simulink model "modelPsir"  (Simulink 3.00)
settings: Solver=ode45  SolverMode=SingleTasking  StartTime=0.0  StopTime=0..5  MaxStep=0.0001  RelTol=1e-5  AbsTol=1e-5
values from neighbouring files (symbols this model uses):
  J = 0.0017    [Data.m]
  kr = Lm/Lr    (= 0.963591022444)    [Data.m]
  Lm = .5796    (= 0.5796)    [Data.m]
  Ls1 = Ls-Lm^2/Lr    (= 0.0430026433915)    [Data.m]
  p = 1    [Data.m]
  R1 = Rs+kr^2*Rr    (= 11.0434783366)    [Data.m]
  T1 = Ls1/R1    (= 0.00389394012293)    [Data.m]
  Tr = Lr/Rr    (= 0.162567567568)    [Data.m]
libraries: simulink_extras x1

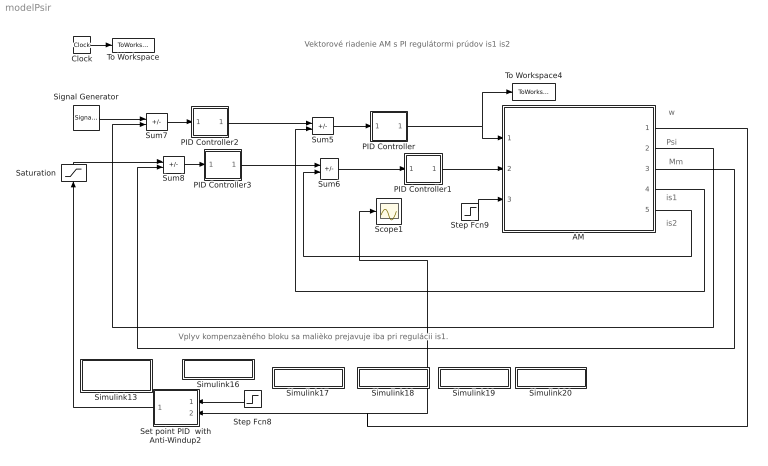
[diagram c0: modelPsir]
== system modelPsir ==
  note: w
  note: Psi
  note: Mm
  note: is1
  note: is2
  note: Vektorové riadenie AM s PI regulátormi prúdov is1 is2
  note: Vplyv kompenzaèného bloku sa malièko prejavuje iba pri regulácii is1.
  AM : Subsystem
  Clock : Clock
  PID Controller : Subsystem  mask(PID Controller){}
      mask help: Enter expressions for proportional, integral, and derivative terms. P+I/s+Ds
      mask init:
      | P=@1; I=@2; D=@3;
  PID Controller1 : Subsystem  mask(PID Controller){}
      mask help: Enter expressions for proportional, integral, and derivative terms. P+I/s+Ds
      mask init:
      | P=@1; I=@2; D=@3;
  PID Controller2 : Subsystem  mask(PID Controller){}
      mask help: Enter expressions for proportional, integral, and derivative terms. P+I/s+Ds
      mask init:
      | P=@1; I=@2; D=@3;
  PID Controller3 : Subsystem  mask(PID Controller){}
      mask help: Enter expressions for proportional, integral, and derivative terms. P+I/s+Ds
      mask init:
      | P=@1; I=@2; D=@3;
  Saturation : Saturate  Orientation=up  UpperLimit=135  LowerLimit=-135
  Scope1 : Scope
  Set point PID  with Anti-Windup2 : Subsystem  Orientation=left  mask(Anti windup PID){}
      mask help: Setpoint PID with anti-windup: e=(ysp-y) P=K*(b*ysp-y) D=(KTds/(1+Td/Ns) dI/dt=(K/Ti)*e+1/Tt(v-u) v=sat(P+I+D)
      mask init:
      | K=@1 ; b =@2 ; Ti=@3 ; Tt=@4 ; ulow=@5(1); uhigh=@5(2); Td=@6(1); N=@6(2);
  Signal Generator : SignalGenerator  WaveForm=sine  Amplitude=1  Frequency=10  Units=Hertz
  Simulink13 : Subsystem
  Simulink16 : Subsystem
  Simulink17 : Subsystem
  Simulink18 : Subsystem
  Simulink19 : Subsystem
  Simulink20 : Subsystem
  Step Fcn8 : Step  Orientation=left  Time=0  Before=0  After=0  SampleTime=-1
  Step Fcn9 : Step  Time=0  Before=0  After=0  SampleTime=-1
  Sum{5..8} (4 alike) : Sum  Inputs=+-  SaturateOnIntegerOverflow=on
  To Workspace : ToWorkspace  VariableName=t  SampleTime=0  SaveFormat=Matrix
  To Workspace4 : ToWorkspace  VariableName=u  SampleTime=0  SaveFormat=Matrix
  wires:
  Clock/1 -> To Workspace/1
  AM/5(out_5) -> Sum6/2
  AM/4(out_4) -> Sum5/2
  Sum5/1 -> PID Controller/1(In_1)
  PID Controller/1(Out_1) -> AM/1(in_1), To Workspace4/1
  Sum6/1 -> PID Controller1/1(In_1)
  PID Controller1/1(Out_1) -> AM/2(in_2)
  Sum7/1 -> PID Controller2/1(In_1)
  AM/2(out_2) -> Sum7/2
  Sum8/1 -> PID Controller3/1(In_1)
  AM/3(out_3) -> Sum8/2
  PID Controller2/1(Out_1) -> Sum5/1
  PID Controller3/1(Out_1) -> Sum6/1
  AM/1(out_1) -> Set point PID  with Anti-Windup2/2(System Output), Scope1/1
  Saturation/1 -> Sum8/1
  Step Fcn9/1 -> AM/3(in_3)
  Step Fcn8/1 -> Set point PID  with Anti-Windup2/1(Set point)
  Set point PID  with Anti-Windup2/1(Input to system) -> Saturation/1
  Signal Generator/1 -> Sum7/1

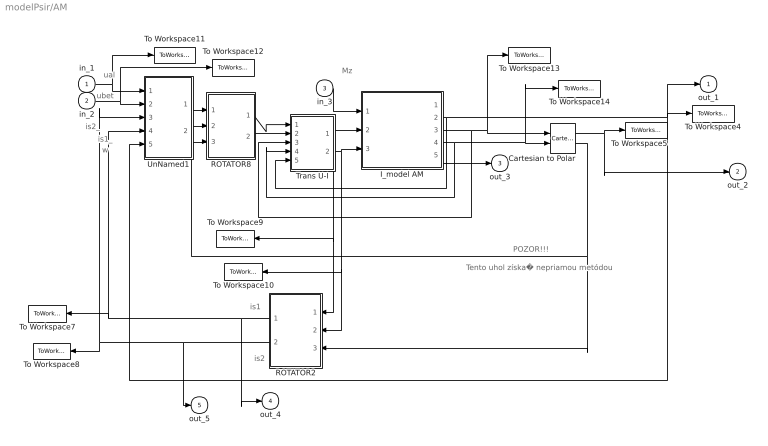
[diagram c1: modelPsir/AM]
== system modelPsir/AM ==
  note: is2_
  note: is1_
  note: w
  note: ubet
  note: ual
  note: Mz
  note: is1
  note: is2
  note: POZOR!!!
  note: Tento uhol získa� nepriamou metódou
  in_1 : Inport  Port=1  PortWidth=-1  SampleTime=-1  DataType=auto
  in_2 : Inport  Port=2  PortWidth=-1  SampleTime=-1  DataType=auto
  in_3 : Inport  Port=3  PortWidth=-1  SampleTime=-1  DataType=auto
  Cartesian to Polar : simulink_extras/Transformations/Cartesian to Polar
  I_model AM : Subsystem
  ROTATOR2 : Subsystem  Orientation=left
  ROTATOR8 : Subsystem
  To Workspace10 : ToWorkspace  VariableName=isb  SampleTime=0  SaveFormat=Matrix
  To Workspace11 : ToWorkspace  VariableName=usal  SampleTime=0  SaveFormat=Matrix
  To Workspace12 : ToWorkspace  VariableName=usb  SampleTime=0  SaveFormat=Matrix
  To Workspace13 : ToWorkspace  VariableName=psisal  SampleTime=0  SaveFormat=Matrix
  To Workspace14 : ToWorkspace  VariableName=psisb  SampleTime=0  SaveFormat=Matrix
  To Workspace4 : ToWorkspace  VariableName=w  SampleTime=0  SaveFormat=Matrix
  To Workspace5 : ToWorkspace  VariableName=Psi  SampleTime=0  SaveFormat=Matrix
  To Workspace7 : ToWorkspace  VariableName=is1  SampleTime=0  SaveFormat=Matrix
  To Workspace8 : ToWorkspace  VariableName=is2  SampleTime=0  SaveFormat=Matrix
  To Workspace9 : ToWorkspace  VariableName=isal  SampleTime=0  SaveFormat=Matrix
  Trans U-I : Subsystem
  UnNamed1 : Subsystem
  out_1 : Outport  Port=1  InitialOutput=0
  out_2 : Outport  Port=2  InitialOutput=0
  out_3 : Outport  Port=3  InitialOutput=0
  out_4 : Outport  Port=4  InitialOutput=0
  out_5 : Outport  Port=5  InitialOutput=0
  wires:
  UnNamed1/2(Outport2) -> ROTATOR8/2(in_2)
  UnNamed1/1(Outport1) -> ROTATOR8/1(in_1)
  Trans U-I/2(out_2) -> I_model AM/3(in_3), To Workspace10/1, ROTATOR2/2(in_2)
  I_model AM/4(out_4) -> Trans U-I/4(in_4), Cartesian to Polar/2, To Workspace14/1
  I_model AM/3(out_3) -> Trans U-I/3(in_6), To Workspace13/1, Cartesian to Polar/1
  ROTATOR8/2(out_2) -> Trans U-I/2(in_2)
  ROTATOR8/1(out_1) -> Trans U-I/1(in_1)
  I_model AM/2(out_2) -> To Workspace4/1, UnNamed1/5(in_5), out_1/1, Trans U-I/5(in_8)
  in_3/1 -> I_model AM/1(in_1)
  Trans U-I/1(out_1) -> I_model AM/2(in_2), To Workspace9/1, ROTATOR2/1(in_1)
  Cartesian to Polar/1 -> To Workspace5/1, out_2/1
  ROTATOR2/1(out_1) -> out_4/1, UnNamed1/4(in_6), To Workspace7/1
  ROTATOR2/2(out_2) -> out_5/1, UnNamed1/3(in_3), To Workspace8/1
  in_1/1 -> UnNamed1/1(in_1), To Workspace11/1
  in_2/1 -> UnNamed1/2(in_2), To Workspace12/1
  I_model AM/5(out_5) -> out_3/1
  Cartesian to Polar/2 -> ROTATOR2/3(in_3), ROTATOR8/3(in_3)

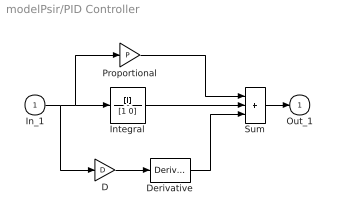
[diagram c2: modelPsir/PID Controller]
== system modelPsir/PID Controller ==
  In_1 : Inport  Port=1  PortWidth=-1  SampleTime=-1  DataType=auto
  D : Gain  Gain=D  SaturateOnIntegerOverflow=on
  Derivative : Derivative
  Integral : TransferFcn  Numerator=[I]  Denominator=[1 0]
  Proportional : Gain  Gain=P  SaturateOnIntegerOverflow=on
  Sum : Sum  Inputs=+++  SaturateOnIntegerOverflow=on
  Out_1 : Outport  Port=1  InitialOutput=0
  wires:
  D/1 -> Derivative/1
  Sum/1 -> Out_1/1
  In_1/1 -> D/1, Integral/1, Proportional/1
  Derivative/1 -> Sum/3
  Integral/1 -> Sum/2
  Proportional/1 -> Sum/1

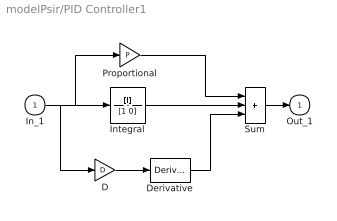
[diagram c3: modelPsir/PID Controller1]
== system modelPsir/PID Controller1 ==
  In_1 : Inport  Port=1  PortWidth=-1  SampleTime=-1  DataType=auto
  D : Gain  Gain=D  SaturateOnIntegerOverflow=on
  Derivative : Derivative
  Integral : TransferFcn  Numerator=[I]  Denominator=[1 0]
  Proportional : Gain  Gain=P  SaturateOnIntegerOverflow=on
  Sum : Sum  Inputs=+++  SaturateOnIntegerOverflow=on
  Out_1 : Outport  Port=1  InitialOutput=0
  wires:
  Proportional/1 -> Sum/1
  Integral/1 -> Sum/2
  Derivative/1 -> Sum/3
  In_1/1 -> Integral/1, Proportional/1, D/1
  Sum/1 -> Out_1/1
  D/1 -> Derivative/1

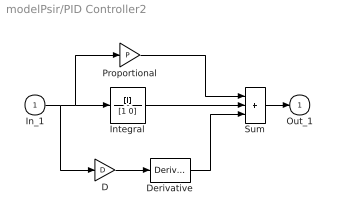
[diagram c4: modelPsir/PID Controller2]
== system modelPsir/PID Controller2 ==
  In_1 : Inport  Port=1  PortWidth=-1  SampleTime=-1  DataType=auto
  D : Gain  Gain=D  SaturateOnIntegerOverflow=on
  Derivative : Derivative
  Integral : TransferFcn  Numerator=[I]  Denominator=[1 0]
  Proportional : Gain  Gain=P  SaturateOnIntegerOverflow=on
  Sum : Sum  Inputs=+++  SaturateOnIntegerOverflow=on
  Out_1 : Outport  Port=1  InitialOutput=0
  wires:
  Proportional/1 -> Sum/1
  Integral/1 -> Sum/2
  Derivative/1 -> Sum/3
  In_1/1 -> Integral/1, Proportional/1, D/1
  Sum/1 -> Out_1/1
  D/1 -> Derivative/1

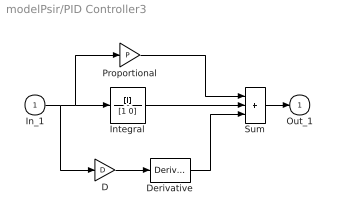
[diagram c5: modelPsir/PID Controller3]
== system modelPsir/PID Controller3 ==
  In_1 : Inport  Port=1  PortWidth=-1  SampleTime=-1  DataType=auto
  D : Gain  Gain=D  SaturateOnIntegerOverflow=on
  Derivative : Derivative
  Integral : TransferFcn  Numerator=[I]  Denominator=[1 0]
  Proportional : Gain  Gain=P  SaturateOnIntegerOverflow=on
  Sum : Sum  Inputs=+++  SaturateOnIntegerOverflow=on
  Out_1 : Outport  Port=1  InitialOutput=0
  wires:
  D/1 -> Derivative/1
  Sum/1 -> Out_1/1
  In_1/1 -> D/1, Integral/1, Proportional/1
  Derivative/1 -> Sum/3
  Integral/1 -> Sum/2
  Proportional/1 -> Sum/1

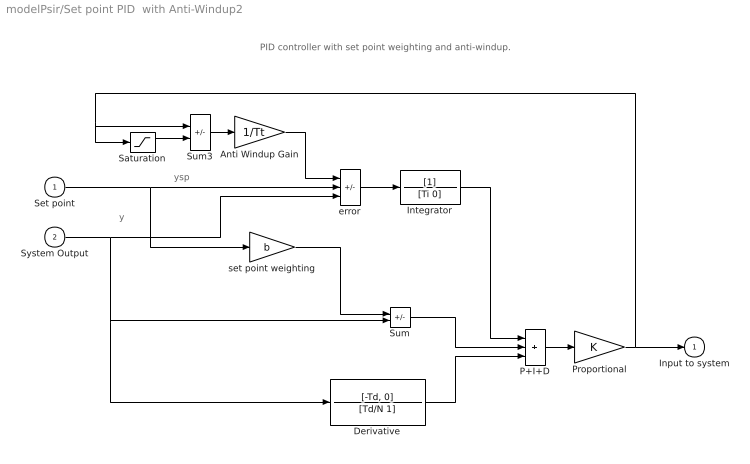
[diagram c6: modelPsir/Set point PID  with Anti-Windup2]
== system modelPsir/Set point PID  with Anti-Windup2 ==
  note: PID controller with set point weighting and anti-windup.
  note: y
  note: ysp
  Set point : Inport  Port=1  PortWidth=-1  SampleTime=-1  DataType=auto
  System Output : Inport  Port=2  PortWidth=-1  SampleTime=-1  DataType=auto
  Anti Windup Gain : Gain  Gain=1/Tt  SaturateOnIntegerOverflow=on
  Derivative : TransferFcn  Numerator=[-Td, 0]  Denominator=[Td/N 1]
  Integrator : TransferFcn  Numerator=[1]  Denominator=[Ti 0]
  P+I+D : Sum  Inputs=+++  SaturateOnIntegerOverflow=on
  Proportional : Gain  Gain=K  SaturateOnIntegerOverflow=on
  Saturation : Saturate  UpperLimit=uhigh  LowerLimit=ulow
  Sum : Sum  Inputs=+-  SaturateOnIntegerOverflow=on
  Sum3 : Sum  Inputs=+-  SaturateOnIntegerOverflow=on
  error : Sum  Inputs=-+-  SaturateOnIntegerOverflow=on
  set point weighting : Gain  Gain=b  SaturateOnIntegerOverflow=on
  Input to system : Outport  Port=1  InitialOutput=0
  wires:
  Integrator/1 -> P+I+D/1
  P+I+D/1 -> Proportional/1
  Derivative/1 -> P+I+D/3
  Sum/1 -> P+I+D/2
  Set point/1 -> error/2, set point weighting/1
  error/1 -> Integrator/1
  Saturation/1 -> Sum3/2
  Sum3/1 -> Anti Windup Gain/1
  Anti Windup Gain/1 -> error/1
  System Output/1 -> error/3, Sum/2, Derivative/1
  Proportional/1 -> Input to system/1, Saturation/1, Sum3/1
  set point weighting/1 -> Sum/1

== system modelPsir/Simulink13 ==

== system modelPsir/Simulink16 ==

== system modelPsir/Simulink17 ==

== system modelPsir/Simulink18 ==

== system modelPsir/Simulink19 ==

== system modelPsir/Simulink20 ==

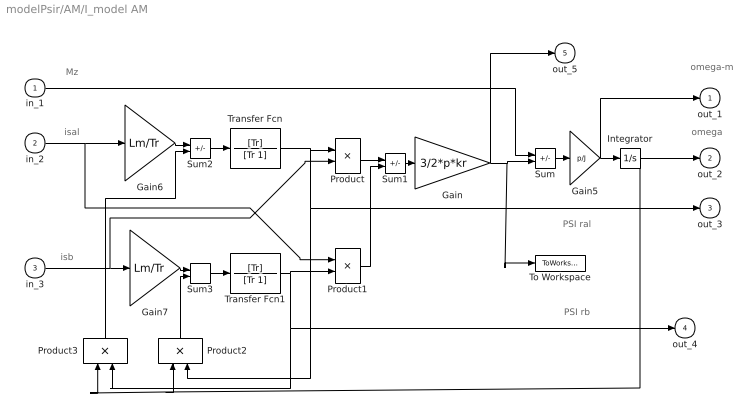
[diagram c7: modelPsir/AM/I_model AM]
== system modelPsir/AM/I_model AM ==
  note: isal
  note: PSI ral
  note: isb
  note: PSI rb
  note: Mz
  note: omega
  note: omega-m
  in_1 : Inport  Port=1  PortWidth=-1  SampleTime=-1  DataType=auto
  in_2 : Inport  Port=2  PortWidth=-1  SampleTime=-1  DataType=auto
  in_3 : Inport  Port=3  PortWidth=-1  SampleTime=-1  DataType=auto
  Gain : Gain  Gain=3/2*p*kr  SaturateOnIntegerOverflow=on
  Gain5 : Gain  Gain=p/J  SaturateOnIntegerOverflow=on
  Gain6 : Gain  Gain=Lm/Tr  SaturateOnIntegerOverflow=on
  Gain7 : Gain  Gain=Lm/Tr  SaturateOnIntegerOverflow=on
  Integrator : Integrator  ExternalReset=none  InitialConditionSource=internal  InitialCondition=0  LimitOutput=off  UpperSaturationLimit=inf  LowerSaturationLimit=-inf  ShowSaturationPort=off  ShowStatePort=off  AbsoluteTolerance=auto
  Product : Product  Inputs=2  SaturateOnIntegerOverflow=on
  Product1 : Product  Inputs=2  SaturateOnIntegerOverflow=on
  Product2 : Product  Orientation=up  Inputs=2  SaturateOnIntegerOverflow=on
  Product3 : Product  Orientation=up  Inputs=2  SaturateOnIntegerOverflow=on
  Sum : Sum  Inputs=-+  SaturateOnIntegerOverflow=on
  Sum1 : Sum  Inputs=+-  SaturateOnIntegerOverflow=on
  Sum2 : Sum  Inputs=+-  SaturateOnIntegerOverflow=on
  Sum3 : Sum  Inputs=++  SaturateOnIntegerOverflow=on
  To Workspace : ToWorkspace  VariableName=Mm  SampleTime=0  SaveFormat=Matrix
  Transfer Fcn : TransferFcn  Numerator=[Tr]  Denominator=[Tr 1]
  Transfer Fcn1 : TransferFcn  Numerator=[Tr]  Denominator=[Tr 1]
  out_1 : Outport  Port=1  InitialOutput=0
  out_2 : Outport  Port=2  InitialOutput=0
  out_3 : Outport  Port=3  InitialOutput=0
  out_4 : Outport  Port=4  InitialOutput=0
  out_5 : Outport  Port=5  InitialOutput=0
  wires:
  Gain/1 -> Sum/2, To Workspace/1, out_5/1
  Product1/1 -> Sum1/2
  in_1/1 -> Sum/1
  in_3/1 -> Gain7/1, Product/2
  Product2/1 -> Sum3/2
  Sum3/1 -> Transfer Fcn1/1
  Sum2/1 -> Transfer Fcn/1
  Product/1 -> Sum1/1
  Sum1/1 -> Gain/1
  Sum/1 -> Gain5/1
  Integrator/1 -> out_2/1, Product3/1, Product2/1
  Transfer Fcn/1 -> Product/1, Product2/2, out_3/1
  Gain5/1 -> Integrator/1, out_1/1
  Gain7/1 -> Sum3/1
  Gain6/1 -> Sum2/1
  Transfer Fcn1/1 -> Product1/2, Product3/2, out_4/1
  Product3/1 -> Sum2/2
  in_2/1 -> Gain6/1, Product1/1

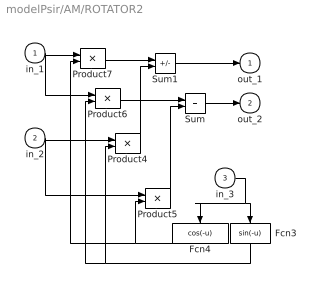
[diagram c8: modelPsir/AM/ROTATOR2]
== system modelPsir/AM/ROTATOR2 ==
  in_1 : Inport  Port=1  PortWidth=-1  SampleTime=-1  DataType=auto
  in_2 : Inport  Port=2  PortWidth=-1  SampleTime=-1  DataType=auto
  in_3 : Inport  Port=3  PortWidth=-1  SampleTime=-1  DataType=auto
  Fcn3 : Fcn  Orientation=down  Expr=sin(-u)
  Fcn4 : Fcn  Orientation=down  Expr=cos(-u)
  Product{4..7} (4 alike) : Product  Inputs=2  SaturateOnIntegerOverflow=on
  Sum : Sum  Inputs=++  SaturateOnIntegerOverflow=on
  Sum1 : Sum  Inputs=+-  SaturateOnIntegerOverflow=on
  out_1 : Outport  Port=1  InitialOutput=0
  out_2 : Outport  Port=2  InitialOutput=0
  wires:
  in_3/1 -> Fcn3/1, Fcn4/1
  in_2/1 -> Product5/1, Product4/1
  Sum/1 -> out_2/1
  Sum1/1 -> out_1/1
  in_1/1 -> Product6/1, Product7/1
  Product4/1 -> Sum1/2
  Product7/1 -> Sum1/1
  Fcn3/1 -> Product4/2, Product6/2
  Product6/1 -> Sum/1
  Product5/1 -> Sum/2
  Fcn4/1 -> Product7/2, Product5/2

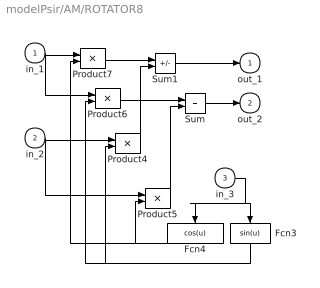
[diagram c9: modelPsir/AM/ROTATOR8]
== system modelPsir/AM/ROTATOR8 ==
  in_1 : Inport  Port=1  PortWidth=-1  SampleTime=-1  DataType=auto
  in_2 : Inport  Port=2  PortWidth=-1  SampleTime=-1  DataType=auto
  in_3 : Inport  Port=3  PortWidth=-1  SampleTime=-1  DataType=auto
  Fcn3 : Fcn  Orientation=down  Expr=sin(u)
  Fcn4 : Fcn  Orientation=down  Expr=cos(u)
  Product{4..7} (4 alike) : Product  Inputs=2  SaturateOnIntegerOverflow=on
  Sum : Sum  Inputs=++  SaturateOnIntegerOverflow=on
  Sum1 : Sum  Inputs=+-  SaturateOnIntegerOverflow=on
  out_1 : Outport  Port=1  InitialOutput=0
  out_2 : Outport  Port=2  InitialOutput=0
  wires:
  Fcn4/1 -> Product7/2, Product5/2
  Product5/1 -> Sum/2
  Product6/1 -> Sum/1
  Fcn3/1 -> Product4/2, Product6/2
  Product7/1 -> Sum1/1
  Product4/1 -> Sum1/2
  in_1/1 -> Product7/1, Product6/1
  Sum1/1 -> out_1/1
  Sum/1 -> out_2/1
  in_2/1 -> Product4/1, Product5/1
  in_3/1 -> Fcn3/1, Fcn4/1

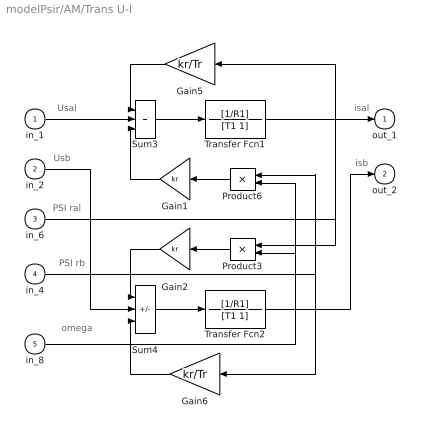
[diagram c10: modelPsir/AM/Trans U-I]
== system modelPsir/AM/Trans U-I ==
  note: PSI rb
  note: PSI ral
  note: omega
  note: Usal
  note: Usb
  note: isal
  note: isb
  in_1 : Inport  Port=1  PortWidth=-1  SampleTime=-1  DataType=auto
  in_2 : Inport  Port=2  PortWidth=-1  SampleTime=-1  DataType=auto
  in_6 : Inport  Port=3  PortWidth=-1  SampleTime=-1  DataType=auto
  in_4 : Inport  Port=4  PortWidth=-1  SampleTime=-1  DataType=auto
  in_8 : Inport  Port=5  PortWidth=-1  SampleTime=-1  DataType=auto
  Gain1 : Gain  Orientation=left  Gain=kr  SaturateOnIntegerOverflow=on
  Gain2 : Gain  Orientation=left  Gain=kr  SaturateOnIntegerOverflow=on
  Gain5 : Gain  Orientation=left  Gain=kr/Tr  SaturateOnIntegerOverflow=on
  Gain6 : Gain  Orientation=left  Gain=kr/Tr  SaturateOnIntegerOverflow=on
  Product3 : Product  Orientation=left  Inputs=2  SaturateOnIntegerOverflow=on
  Product6 : Product  Orientation=left  Inputs=2  SaturateOnIntegerOverflow=on
  Sum3 : Sum  Inputs=+++  SaturateOnIntegerOverflow=on
  Sum4 : Sum  Inputs=-++  SaturateOnIntegerOverflow=on
  Transfer Fcn1 : TransferFcn  Numerator=[1/R1]  Denominator=[T1 1]
  Transfer Fcn2 : TransferFcn  Numerator=[1/R1]  Denominator=[T1 1]
  out_1 : Outport  Port=1  InitialOutput=0
  out_2 : Outport  Port=2  InitialOutput=0
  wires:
  in_2/1 -> Sum4/2
  Gain1/1 -> Sum3/3
  Gain2/1 -> Sum4/1
  Transfer Fcn2/1 -> out_2/1
  Transfer Fcn1/1 -> out_1/1
  Sum3/1 -> Transfer Fcn1/1
  Sum4/1 -> Transfer Fcn2/1
  Gain6/1 -> Sum4/3
  Gain5/1 -> Sum3/1
  in_1/1 -> Sum3/2
  Product6/1 -> Gain1/1
  Product3/1 -> Gain2/1
  in_8/1 -> Product6/2, Product3/2
  in_6/1 -> Product3/1, Gain5/1
  in_4/1 -> Gain6/1, Product6/1

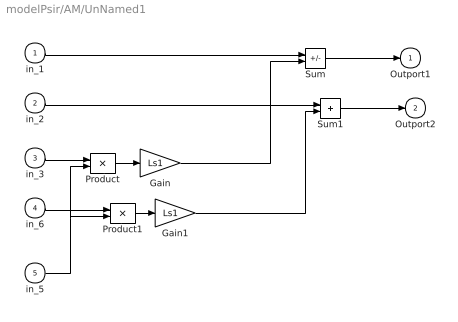
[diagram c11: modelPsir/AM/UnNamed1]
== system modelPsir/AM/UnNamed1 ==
  in_1 : Inport  Port=1  PortWidth=-1  SampleTime=-1  DataType=auto
  in_2 : Inport  Port=2  PortWidth=-1  SampleTime=-1  DataType=auto
  in_3 : Inport  Port=3  PortWidth=-1  SampleTime=-1  DataType=auto
  in_6 : Inport  Port=4  PortWidth=-1  SampleTime=-1  DataType=auto
  in_5 : Inport  Port=5  PortWidth=-1  SampleTime=-1  DataType=auto
  Gain : Gain  Gain=Ls1  SaturateOnIntegerOverflow=on
  Gain1 : Gain  Gain=Ls1  SaturateOnIntegerOverflow=on
  Product : Product  Inputs=2  SaturateOnIntegerOverflow=on
  Product1 : Product  Inputs=2  SaturateOnIntegerOverflow=on
  Sum : Sum  Inputs=+-  SaturateOnIntegerOverflow=on
  Sum1 : Sum  Inputs=++  SaturateOnIntegerOverflow=on
  Outport1 : Outport  Port=1  InitialOutput=0
  Outport2 : Outport  Port=2  InitialOutput=0
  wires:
  Sum1/1 -> Outport2/1
  in_2/1 -> Sum1/1
  Gain1/1 -> Sum1/2
  Product1/1 -> Gain1/1
  in_5/1 -> Product/2, Product1/2
  in_6/1 -> Product1/1
  Sum/1 -> Outport1/1
  Gain/1 -> Sum/2
  in_1/1 -> Sum/1
  Product/1 -> Gain/1
  in_3/1 -> Product/1
